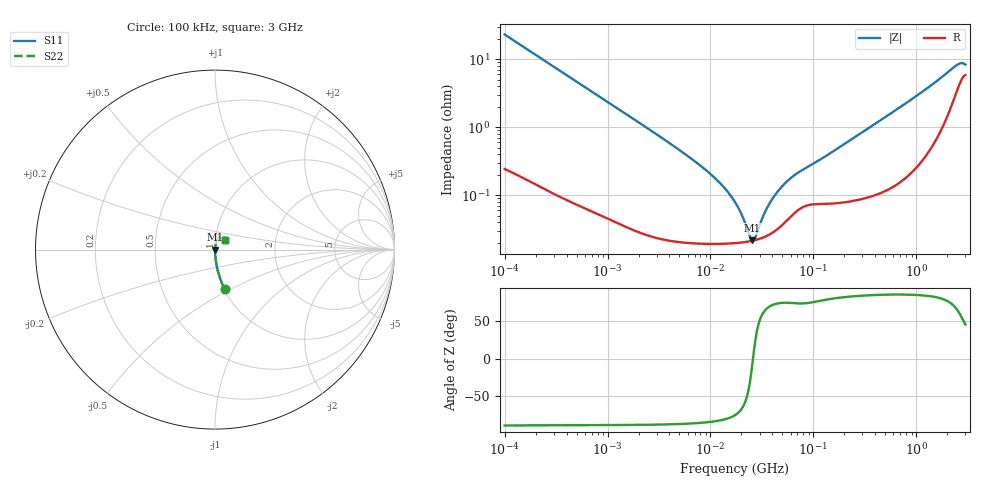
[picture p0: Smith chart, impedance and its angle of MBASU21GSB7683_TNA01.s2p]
! MBASU21GSB7683_TNA01  S-PARAMETER MODEL  ( Standard Model )
! Model Generated by TAIYO YUDEN Corporation (http://www.ty-top.com)
! Version 1.0
! TAIYO YUDEN Control No. 220601
! Copyright(c) 2018 TAIYO YUDEN CO.,LTD. All Rights Reserved.
! Product Description (link to TY-COMPAS)
! https://ds.yuden.co.jp/TYCOMPAS/or/detail?pn=MBASU21GSB7683KTNA01&u=M
! Products Name : Multilayer Ceramic Capacitors
! Characteristics :
!  Capacitance : 0.068 [uF] , Rated Voltage : 50 [V] , TCC : X7R
!  Case Size : 2.0 x 1.25 / 0.079 x 0.049 [mm/inch] , Thickness : 1.25 / 0.049 [mm/inch]
!  (Conditions: Temperature = 25 [degC] , DC Bias Voltage = 0 [V])
! External Node Assignments :
!  1  o---| |---o  2
! GND o---------o GND
! Frequency Range : 100kHz  -  3GHz  [ 401 STEP ]
# MHZ S RI R 50
! Freq[MHz].  S11 Real  S11 Imag  S21 Real  S21 Imag  S12 Real  S12 Imag  S22 Real  S22 Imag
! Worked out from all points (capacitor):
!   401 points, 100 kHz to 3 GHz, reference 50 ohm
!   read as one part in series: C = 68.4 nF near 105.3 kHz
!   lowest |Z| = 21.4 mohm at 25.49 MHz (marker M1)
!   series resonance near 25.91 MHz, so ESL is about 550 pH
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0.1  0.0532 -0.2193  0.9468 0.2193  0.9468 0.2193  0.0532 -0.2193
0.222319  0.0122 -0.1036  0.9878 0.1036  0.9878 0.1036  0.0122 -0.1036
0.562235  0.00241 -0.0417  0.9976 0.0417  0.9976 0.0417  0.00241 -0.0417
3.161081  0.000283 -0.00743  0.9997 0.00743  0.9997 0.00743  0.000283 -0.00743
6.3393  0.000208 -0.00354  0.9998 0.00354  0.9998 0.00354  0.000208 -0.00354
10.08119  0.000195 -0.00201  0.9998 0.00201  0.9998 0.00201  0.000195 -0.00201
14.09348  0.000194 -0.0012  0.9998 0.0012  0.9998 0.0012  0.000194 -0.0012
17.7727  0.000197 -0.000714  0.9998 0.000714  0.9998 0.000714  0.000197 -0.000714
20.21703  0.0002 -0.000464  0.9998 0.000464  0.9998 0.000464  0.0002 -0.000464
24.21403  0.000209 -0.000126  0.9998 0.000126  0.9998 0.000126  0.000209 -0.000126
25.49486  0.000212 -2.97e-05  0.9998 2.97e-05  0.9998 2.97e-05  0.000212 -2.97e-05
27.54426  0.000218 0.000114  0.9998 -0.000114  0.9998 -0.000114  0.000218 0.000114
32.15051  0.000236 0.000406  0.9998 -0.000406  0.9998 -0.000406  0.000236 0.000406
35.64176  0.000253 0.000606  0.9997 -0.000606  0.9997 -0.000606  0.000253 0.000606
44.94634  0.000318 0.00108  0.9997 -0.00108  0.9997 -0.00108  0.000318 0.00108
62.83488  0.000514 0.0018  0.9995 -0.0018  0.9995 -0.0018  0.000514 0.0018
97.38194  0.000735 0.00273  0.9993 -0.00273  0.9993 -0.00273  0.000735 0.00273
547.5153  0.00146 0.0154  0.9985 -0.0154  0.9985 -0.0154  0.00146 0.0154
1217.231  0.00487 0.0351  0.9951 -0.0351  0.9951 -0.0351  0.00487 0.0351
2378.954  0.0328 0.0692  0.9672 -0.0692  0.9672 -0.0692  0.0328 0.0692
2706.139  0.0501 0.0668  0.9499 -0.0668  0.9499 -0.0668  0.0501 0.0668
3000  0.0583 0.053  0.9417 -0.053  0.9417 -0.053  0.0583 0.053
